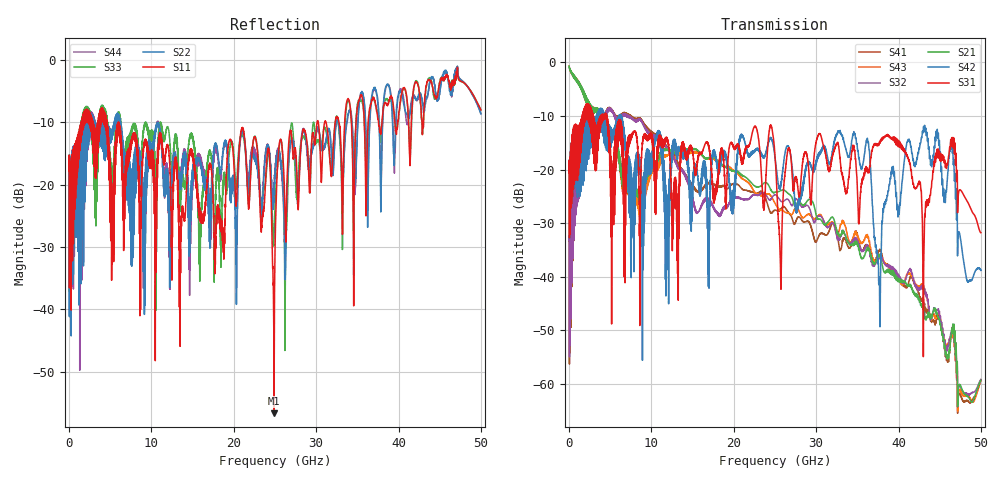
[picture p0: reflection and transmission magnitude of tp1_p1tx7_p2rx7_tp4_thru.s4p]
! 100G CR Analysis
! File: tp1_p1tx7_p2rx7_tp4_thru
! Description: 2m Cu Cable, OSFP, TP1-TP4
! Port Mapping
! Port1 -- P1TX7N
! Port2 -- P2RX7N
! Port3 -- P1TX7P
! Port4 -- P2RX7P
# GHz S MA R 50.00
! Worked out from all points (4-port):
!   5000 points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, 10 MHz to 50 GHz, reference 50 ohm
!   strongest paths, dB at 10 MHz, 12.51 GHz, 25.01 GHz, 37.51 GHz, 50 GHz:
!     S31: -20.5, -27.3, -17.5, -15.5, -31.8
!     S42: -20.5, -15.9, -17.8, -36.7, -38.8
!     S21: -0.7, -16.8, -24.2, -36.3, -59.3
!     S32: -33.2, -17.3, -24.7, -36.8, -59.2
!     S43: -0.7, -17.8, -26.3, -36.9, -59.2
!     S41: -33.3, -16.7, -27.6, -35.7, -59.4
!   lowest |S11| = -56.7 dB at 24.88 GHz (marker M1), VSWR 1.00, Z = 50.1 + j0.0849 ohm
!   |S11| at or under -10 dB: start of sweep to 1.489 GHz; 4.584 GHz to 6.019 GHz (1.435 GHz wide, 27.1 % of centre); 6.021 GHz to 30.11 GHz (24.09 GHz wide, 133 % of centre)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
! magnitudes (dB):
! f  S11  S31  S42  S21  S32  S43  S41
! 10 MHz  -17.8  -20.5  -20.5  -0.7  -33.2  -0.7  -33.3
! 4.89 GHz  -19.3  -16.0  -16.5  -13.7  -8.6  -13.8  -8.5
! 24.88 GHz  -56.7  -15.1  -16.3  -24.3  -24.8  -25.9  -27.6
! 25.66 GHz  -12.7  -37.5  -23.4  -24.0  -25.8  -27.6  -27.5
! 37.65 GHz  -10.6  -15.3  -41.5  -36.1  -36.6  -36.7  -35.3
! 43.21 GHz  -5.6  -28.9  -12.9  -47.9  -43.1  -43.2  -46.2
! 50 GHz  -8.0  -31.8  -38.8  -59.3  -59.2  -59.2  -59.4
